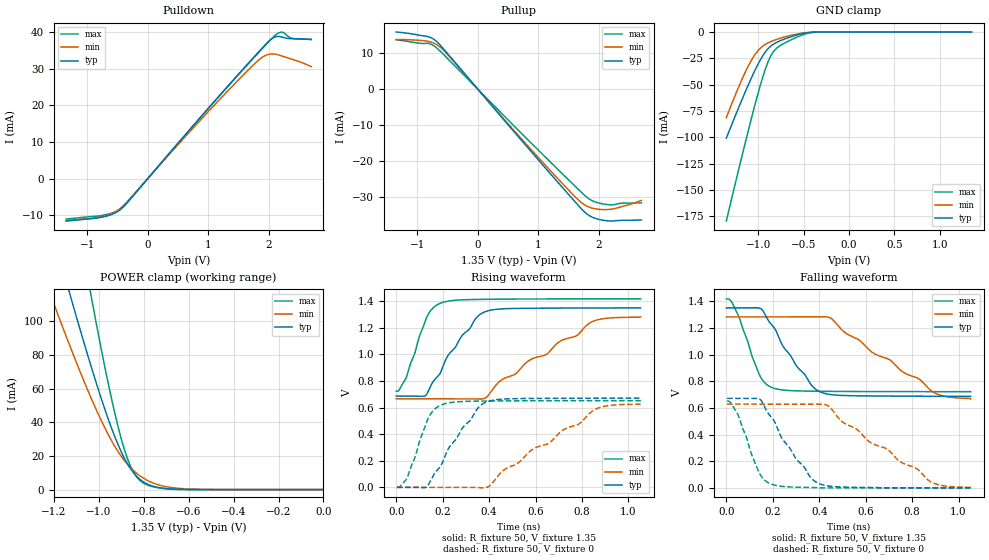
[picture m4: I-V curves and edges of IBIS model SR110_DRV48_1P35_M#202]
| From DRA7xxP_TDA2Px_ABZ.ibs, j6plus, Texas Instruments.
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| Model based on original model for DDR_DIFFIOPB_H
|   Sub model SR110_DRV48_1P35
[model]   SR110_DRV48_1P35_M#202
|[Description]  [1.35V-I/O-X-X]
|   , ,
|[Input Load]
|[Output Drive]
|Voltage   1.35V
|Mode   I/O
Model_type   I/O
Polarity   Non-Inverting
Enable   Active-Low
Vinl =  0.585
Vinh =  0.765
Cref =  15.0000pF
Rref =  100.0000M
Vref =  0V
Vmeas =  0.675
C_comp   2p   2p   2p
[Model Spec]
Vinl   0.585   0.55125   0.61875
Vinh   0.765   0.73125   0.79875
[Receiver Thresholds]
Tslew_ac = 5n
Vth = 0.675
Vth_max = 0.709
Vth_min = 0.608
Vinh_ac = 0.175
Vinh_dc = 0.1
Vinl_ac = -0.175
Vinl_dc = -0.1
[Temperature Range]   25   125   -40
[Voltage Range]   1.35   1.2825   1.4175
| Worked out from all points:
|   slope of the pulldown table from 0 to 0.203 V, typ, clamps not added: 51.5 ohm
|   slope of the pullup table from 0 to 0.203 V, typ, clamps not added: 50.4 ohm
|   GND clamp passes 1 mA (typ) near -0.48 V on its own axis
|   POWER clamp passes 1 mA (typ) near -0.72 V on its own axis
|   rising waveform, R_fixture 50, V_fixture 1.35: 20-80 % time 154ps typ, 349ps min, 81.4ps max; typ from 0.687 V to 1.35 V
|   rising waveform, R_fixture 50, V_fixture 0: 20-80 % time 151ps typ, 343ps min, 79.7ps max; typ from 0 V to 0.671 V
|   falling waveform, R_fixture 50, V_fixture 1.35: 20-80 % time 151ps typ, 332ps min, 83.7ps max; typ from 1.35 V to 0.687 V
|   falling waveform, R_fixture 50, V_fixture 0: 20-80 % time 153ps typ, 337ps min, 80.2ps max; typ from 0.671 V to 0 V
[POWER_clamp]
-1.35V    224.4mA    165.8mA    358.5mA
-1.214V   157mA      115.5mA    250.8mA
-1.132V   117.8mA    86.59mA    187.7mA
-1.118V   111.4mA    81.92mA    177.3mA
-1.036V   74.26mA    55.16mA    116.8mA
-954.5mV  40.7mA     31.91mA    61.06mA
-900mV    22.42mA    19.79mA    30.14mA
-859.1mV  12.48mA    13.09mA    13.96mA
-804.5mV  4.85mA     7.084mA    4.132mA
-736.4mV  1.313mA    2.9mA      1.073mA
-627.3mV  101.6uA    577.3uA    45.9uA
0V        75.63nA    322.4nA    418.5nA
[Pulldown]
-1.35V    -11.61mA   -11.5mA    -11.06mA
-736.4mV  -10.48mA   -10.33mA   -10.03mA
-531.8mV  -9.35mA    -9.062mA   -9.043mA
-409.1mV  -7.817mA   -7.49mA    -7.751mA
1.145V    21.94mA    20.88mA    21.88mA
1.718V    32.55mA    30.62mA    32.41mA
1.923V    36.25mA    33.48mA    36.08mA
2.005V    37.61mA    33.98mA    37.53mA
2.086V    38.57mA    34.03mA    38.89mA
2.209V    38.7mA     33.51mA    40.04mA
2.373V    38.22mA    32.66mA    38.36mA
2.7V      37.95mA    30.56mA    38.05mA
[Pullup]
-1.35V    15.95mA    13.86mA    13.81mA
-981.8mV  15.11mA    13.66mA    12.86mA
-818.2mV  14.65mA    13.35mA    12.79mA
-736.4mV  14.02mA    12.92mA    12.23mA
-613.6mV  12.13mA    11.6mA     10.47mA
1.064V    -20.91mA   -20.19mA   -18.01mA
1.555V    -30.35mA   -29.03mA   -26.14mA
1.759V    -34.1mA    -32.12mA   -29.45mA
1.923V    -35.82mA   -33.22mA   -31.26mA
2.168V    -36.64mA   -33.43mA   -32.13mA
2.414V    -36.45mA   -32.48mA   -31.67mA
2.7V      -36.37mA   -30.94mA   -31.63mA
[GND_clamp]
-1.35V    -100.7mA   -81.27mA   -179.3mA
-1.241V   -77.31mA   -57.61mA   -140mA
-1.132V   -54.83mA   -36.31mA   -101.6mA
-1.05V    -39.08mA   -23.36mA   -74mA
-968.2mV  -25.28mA   -14.71mA   -48.34mA
-913.6mV  -18.13mA   -11.32mA   -33.52mA
-859.1mV  -13.28mA   -9.024mA   -22.35mA
-831.8mV  -11.61mA   -8.091mA   -18.64mA
-777.3mV  -9.078mA   -6.444mA   -14.07mA
-531.8mV  -1.871mA   -1.307mA   -3.441mA
-368.2mV  -88.76uA   -111.2uA   -158uA
1.35V     75.63nA    385.5nA    349.4nA
[Ramp]
dV/dt_f 0.39869864/0.1509044n 0.37093523/0.33253033n  0.4179992/83.842316p
dV/dt_r 0.40473715/0.15265264n 0.37924418/0.3449013n  0.3922979/79.856587p
R_load = 50
[Rising Waveform]
R_fixture = 50
V_fixture = 1.35
V_fixture_min = 1.2825
V_fixture_max = 1.4175
0s        686.6mV    666.1mV    722.7mV
43.16ps   686mV      666.1mV    825.3mV
124.3ps   688.2mV    666mV      1.248V
152ps     774.7mV    666mV      1.337V
193.6ps   873.8mV    666.1mV    1.387V
281.6ps   1.137V     665.8mV    1.41V
389.8ps   1.325V     679.7mV    1.414V
450.9ps   1.342V     804.3mV    1.415V
838.5ps   1.349V     1.241V     1.417V
1.053ns   1.35V      1.282V     1.417V
[Rising Waveform]
R_fixture = 50
V_fixture = 0
V_fixture_min = 0
V_fixture_max = 0
3.131ps   0V         0V         0V
46.85ps   0V         0V         71.09mV
130.3ps   0V         0V         488.4mV
159.3ps   89.14mV    0V         577.3mV
201.5ps   196.6mV    0V         624.9mV
286.8ps   449.9mV    0V         645.6mV
395.4ps   646.1mV    3.783mV    649.6mV
581.7ps   668.7mV    279.3mV    651.2mV
855.6ps   670.7mV    585.1mV    651.7mV
1.056ns   671.4mV    628.3mV    651.8mV
[Falling Waveform]
R_fixture = 50
V_fixture = 1.35
V_fixture_min = 1.2825
V_fixture_max = 1.4175
0s        1.35V      1.282V     1.417V
20.94ps   1.35V      1.283V     1.4V
52.66ps   1.35V      1.283V     1.291V
145.6ps   1.347V     1.283V     837.4mV
199.1ps   1.216V     1.283V     750.7mV
303.9ps   911.1mV    1.282V     727.6mV
412.4ps   714.4mV    1.284V     724.3mV
452.2ps   699.3mV    1.27V      723.8mV
896.3ps   687.5mV    713.5mV    721.9mV
1.053ns   686.6mV    666.1mV    721.8mV
[Falling Waveform]
R_fixture = 50
V_fixture = 0
V_fixture_min = 0
V_fixture_max = 0
3.131ps   671.4mV    628.3mV    651.8mV
50.91ps   671.6mV    628.3mV    546mV
141.5ps   667.6mV    628.4mV    112.2mV
197.2ps   523.6mV    628.3mV    25.77mV
298.9ps   221.6mV    628.3mV    4.847mV
367.2ps   69.86mV    628.3mV    2.459mV
405.9ps   27.45mV    628.2mV    0V
439.9ps   13.77mV    613.9mV    0V
882.1ps   0V         43.73mV    0V
1.056ns   0V         0V         0V
